(* Logix 5000 AddOnInstructionDefinition export Banner_LM_Param_v4; software revision 33.00 *)

TYPE Banner_IOL_Port_v4 :   // UDT that has all of the data items necessary to communicate with a specific Port on a IO-Link Master
STRUCT
   Port_Controlled : INT;   // Each bit represents a port on an IO-Link Master. Set to 1 to tell AOI to control that port.
   Port_Activate : INT;   // Each bit represents a port on an IO-Link Master. When ON that port will process any commands in queue.
   Port_Read : INT;   // Each bit represents a port on an IO-Link Master. Used to determine when device AOI has requested a Read command.
   Port_Write : INT;   // Each bit represents a port on an IO-Link Master. Used to determine when device AOI has requested a Write command.
   Port_RW_Complete : INT;   // Each bit represents a port on an IO-Link Master. Tells device AOI that Read or Write request has been completed.
   Port_Device_Read : INT;
   Data_Transfer : SINT[190];   // Array to transfer data from IO-Master to device AOIs.
END_STRUCT
END_TYPE

TYPE Banner_LM_RD_v4 :   // UDT that stores the Write Data for a LM.
STRUCT
   Master_Cycle_Time : INT;
   Min_Cycle_Time : INT;
   M_Sequence_Capability : INT;
   IO_Link_Version_ID : INT;
   Process_Data_Input_Length : INT;
   Process_Data_Output_Length : INT;
   Combined_Vendor_ID : DINT;   // IO-Link Vendor ID
   Vendor_ID1 : INT;
   Vendor_ID2 : INT;
   Combined_Device_ID : DINT;   // IO-Link Device ID
   Device_ID1 : INT;
   Device_ID2 : INT;
   Device_ID3 : INT;
   Serial_Number : STRING;
   Teach_State : SINT;   // 0 =IDLE, 1 = SP1 Success, 4 = Wait for Command, 5 = Busy, 7 = Error
   SP1_TP1 : SINT;
   SP2_TP2 : SINT;
   Measurement_Distance : DINT;   // Current measured distance in micrometers.
   Excess_Gain_Percent : DINT;   // Excess gain expressed as a percentage of minimum signal strength.
   Stability : INT;   // 0 = No target exists, 1 = Marginal or multiple peaks, 2 = Stable
   Laser_Fault_Status : INT;   // 0 = Not present, 1 Laser fault present
   Analog_Output_Value : DINT;   // In .01 microAmp increments.
   BDC1_Dual_Mode_Percent : DINT;   // In .01% increments.
   Temperature : INT;
   Last_Taught_Temperature : INT;
   Transducer_Disable_Status : SINT;   // 0 = Active, 1 = Inactive
   All_Time_Run_Time : DINT;   // Run Counter in 1/4 hr increments
   Display_String_Line_1 : STRING;   // String currently being displayed on the LED display of the sensor
   Display_String_Line_2 : STRING;   // String currently being displayed on the LED display of the sensor
   All_Time_Run_Time_Event_Time : DINT;   // Event Time in 1/4 hr increments
END_STRUCT
END_TYPE

TYPE Banner_LM_v4 :   // All of the parameters for a LM.
STRUCT
   Initial_Global_Read : BOOL;   // Determines if all of the IO-Link data has been read into the PLC yet
   Command : INT;   // Value placed in here will activate a read or write to a specifc IO-Link Index
   Read_Data : Banner_LM_RD_v4;   // Read Only Data
   Write_Data : Banner_LM_WD_v4;   // Write Data
   Archive : Banner_LM_WD_v4;   // Archive of Write Data
   Reset : BOOL;   // Resets AOI. This will force a complete parameter read of the sensor.
END_STRUCT
END_TYPE

TYPE Banner_LM_WD_v4 :   // UDT that stores the Write Data for a LM.
STRUCT
   System_Command : INT;   // See IODD file for list of commands that can be activated via the System Command interface
   Parameter_Access_Lock : SINT;   // Write access to all parameters is prohibited while value is 1. Only this parameter can be adjusted when value is 1.
   Data_Storage_Lock : SINT;   // Automatic data storage is disabled when this value is equal to 1. Read access is not affected.
   Local_Parameterization_Lock : SINT;   // Parameterization via local control elements on device is disabled.
   Local_User_Interface_Lock : SINT;   // Operation of local user interface is disabled.
   Teach_Channel : INT;   // 0 = Default, 1 = BDC1, 192 = AO1
   BDC1_Setpoint_SP1 : DINT;   // Switch point value in micrometers. Range: varies depending on sensor.
   BDC1_Setpoint_SP2 : DINT;   // Switch point 2 in window mode only. Range varies depending on sensor.
   BDC1_Swithpoint_Logic : INT;   // 0 = Light Operate, 1 = Dark Operate
   BDC1_BDC_Mode : INT;   // 1 = Switch Mode/Single Point, 2 = Window Mode, 131 = Dual, 132 = Health (LO)/Alarm (DO)
   BDC1_Hysteresis : DINT;   // Should always be 0
   Response_Speed : INT;   // 0 = Fast ms, 1 = Standard, 2 = Medium, 3 = Slow
   Zero_Reference_Location : INT;   // 0 = Near, 1 = Far
   Shift_Zero_Reference_After_Teach : INT;   // 0 = Off, 1 = AutoSet, 2 = SetZero
   Sensor_Lockout : INT;   // 0 =No Lock-out, 1 = Sensor Locked
   Output_Polarity : INT;   // 0 = PNP, 1 = NPN
   IOL_Filter_Time : DINT;   // Time to average IOL process data measurement between updates. Range 0 to 65535 ms.
   Display_Units : SINT;   // 0 = mm, 1 = inches
   Remote_Input_Types : SINT;   // 0 = Type Teach, 1 = Type Laser Enable, 2 = Type Trigger, 3 = Type Sync Master, 4 = Type Sync Slave, 5 = Type Disabled
   Process_Data_Measurement_1_Selection : SINT;   // 0 = Disabled, 1 = Distance Measurement Value, 2 = Displayed Distance Measurement Value, 3 = Analog Output Value, 4 = BDC1 Dual Mode Percent
   Process_Data_Measurement_2_Selection : SINT;   // 0 = Disabled, 1 = Excess Gain, 2 = ExcessGain/10, 3= BDC1 Dual Mode Percent.
   Include_Binary_in_PDI : SINT;   // 0 = Don't include, 1 = Include
   BDC1_Delay_Mode : INT;   // 0 = Disabled, 1 = On - Off Delay, 2 = Off Oneshot, 3 = On Oneshot
   BDC1_Delay_On : DINT;   // Range 0 to 9999 in ms.
   BDC1_Delay_Off : DINT;   // Range 0 to 9999 in ms.
   Swtich_Point_Reference : SINT;   // 0 = Object, 1 = Background, 2= Custom
   User_Teach_Offset : DINT;   // Range -90000 to 90000. User selected teach offset.
   Midpoint_Teach_Window_Size : DINT;   // Range 1000 to 90000. Only used in window mode teach.
   Midpoint_Teach_Offset_Size : DINT;   // Range -90000 to 90000. Offset value that is applied to a midpoint teach.
   BDC_Auto_Thresholding : SINT;   // 0 = On, 1 = Off, 2 = High Speed
   Resettable_Run_Time : DINT;   // Run Counter in 1/4 hr increments
   Resettable_Run_Time_Event_Time : DINT;   // Event Time in 1/4 hour increments
END_STRUCT
END_TYPE

ADD_ON_INSTRUCTION Banner_LM_Param_v4   (* revision 4.1, vendor Banner Engineering *)
// AOI to read and write parameter data to an IO-Link LM.
VAR_IN_OUT
   LM : Banner_LM_v4; {required}
   Port_Data : Banner_IOL_Port_v4; {required}
END_VAR
VAR_INPUT
   Port : INT; {required}
END_VAR
VAR
   Local_Control : DINT; {access None}
   Global_Read_Command_Value : INT; {access None}
   Global_Write_Command_Value : INT; {access None}
   Command_Being_Processed : BOOL; {access None}
   Update_Archive : BOOL; {access None}
   Index_Write_Inprocess : INT; {access None}
   Index_Write_Control : INT; {access None}
   Temp_Excess_Gain : DINT; {access None}
   Inprocess_Index : DINT; {access None}
END_VAR

ROUTINE Logic   (* ladder *)
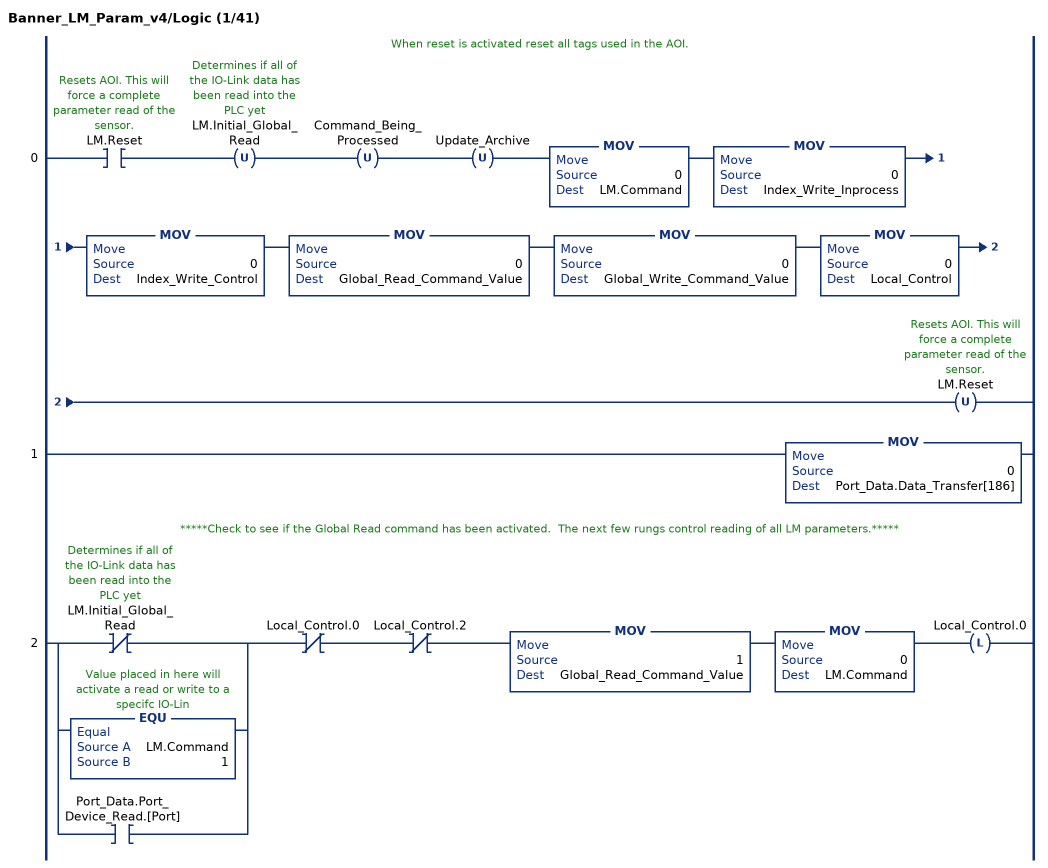
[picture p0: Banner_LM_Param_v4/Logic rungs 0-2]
   // When reset is activated reset all tags used in the AOI.
   0: XIC(LM.Reset)OTU(LM.Initial_Global_Read)OTU(Command_Being_Processed)OTU(Update_Archive)MOV(0,LM.Command)MOV(0,Index_Write_Inprocess)MOV(0,Index_Write_Control)MOV(0,Global_Read_Command_Value)MOV(0,Global_Write_Command_Value)MOV(0,Local_Control)OTU(LM.Reset);
   1: MOV(0,Port_Data.Data_Transfer[186]);
   // *****Check to see if the Global Read command has been activated.  The next few rungs control reading of all LM parameters.*****
   2: [XIO(LM.Initial_Global_Read) ,EQU(LM.Command,1) ,XIC(Port_Data.Port_Device_Read.[Port]) ]XIO(Local_Control.0)XIO(Local_Control.2)MOV(1,Global_Read_Command_Value)MOV(0,LM.Command)OTL(Local_Control.0);
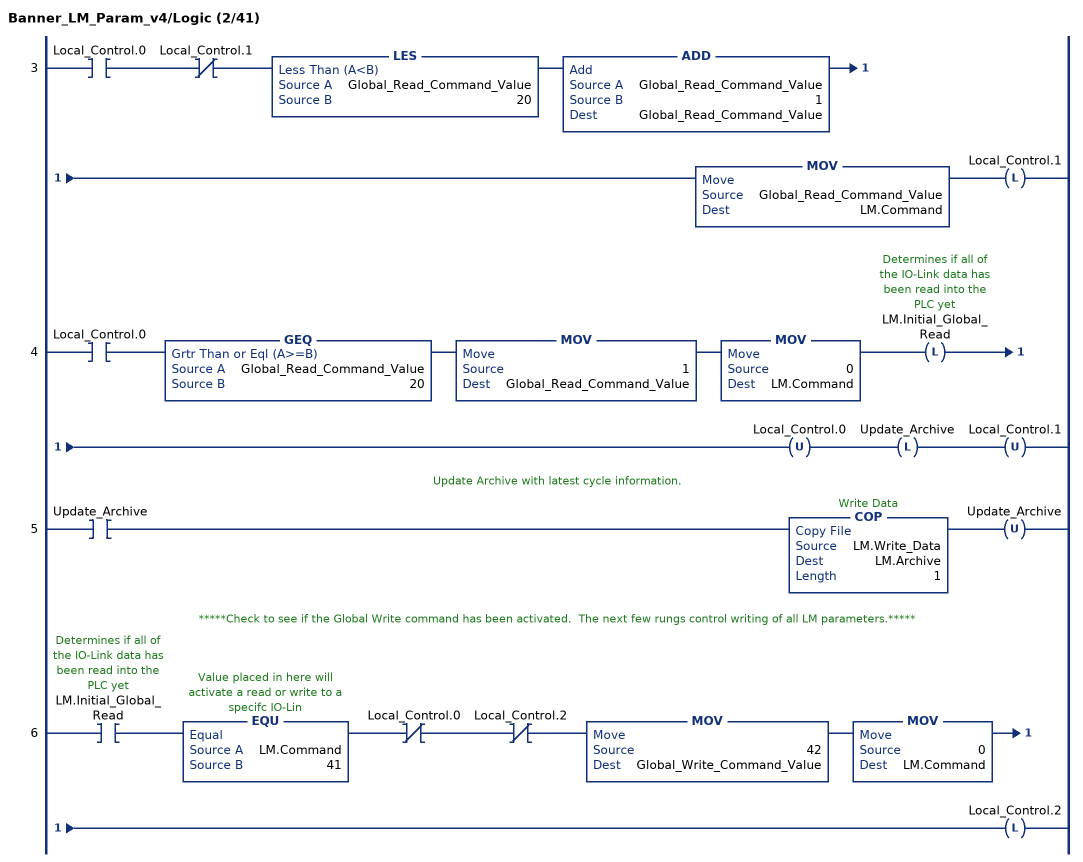
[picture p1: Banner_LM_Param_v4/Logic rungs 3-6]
   3: XIC(Local_Control.0)XIO(Local_Control.1)LES(Global_Read_Command_Value,20)ADD(Global_Read_Command_Value,1,Global_Read_Command_Value)MOV(Global_Read_Command_Value,LM.Command)OTL(Local_Control.1);
   4: XIC(Local_Control.0)GEQ(Global_Read_Command_Value,20)MOV(1,Global_Read_Command_Value)MOV(0,LM.Command)OTL(LM.Initial_Global_Read)OTU(Local_Control.0)OTL(Update_Archive)OTU(Local_Control.1);
   // Update Archive with latest cycle information.
   5: XIC(Update_Archive)COP(LM.Write_Data,LM.Archive,1)OTU(Update_Archive);
   // *****Check to see if the Global Write command has been activated.  The next few rungs control writing of all LM parameters.*****
   6: XIC(LM.Initial_Global_Read)EQU(LM.Command,41)XIO(Local_Control.0)XIO(Local_Control.2)MOV(42,Global_Write_Command_Value)MOV(0,LM.Command)OTL(Local_Control.2);
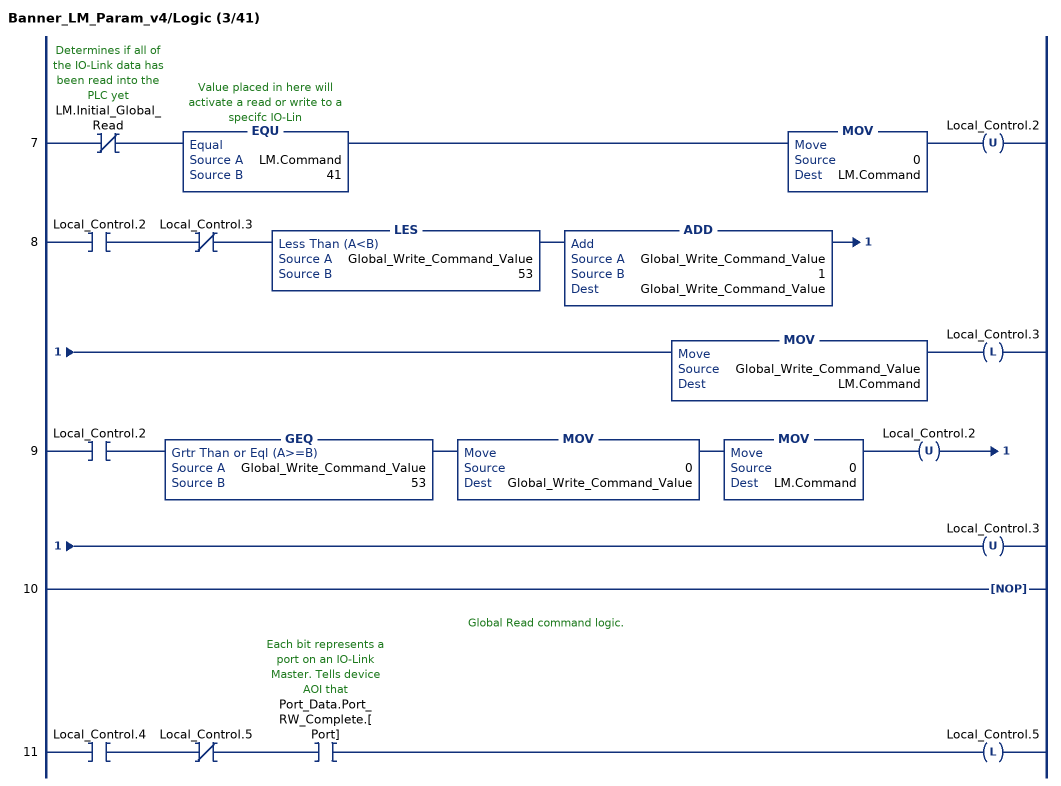
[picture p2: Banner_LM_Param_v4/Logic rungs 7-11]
   7: XIO(LM.Initial_Global_Read)EQU(LM.Command,41)MOV(0,LM.Command)OTU(Local_Control.2);
   8: XIC(Local_Control.2)XIO(Local_Control.3)LES(Global_Write_Command_Value,53)ADD(Global_Write_Command_Value,1,Global_Write_Command_Value)MOV(Global_Write_Command_Value,LM.Command)OTL(Local_Control.3);
   9: XIC(Local_Control.2)GEQ(Global_Write_Command_Value,53)MOV(0,Global_Write_Command_Value)MOV(0,LM.Command)OTU(Local_Control.2)OTU(Local_Control.3);
   10: NOP();
   // Global Read command logic.
   11: XIC(Local_Control.4)XIO(Local_Control.5)XIC(Port_Data.Port_RW_Complete.[Port])OTL(Local_Control.5);
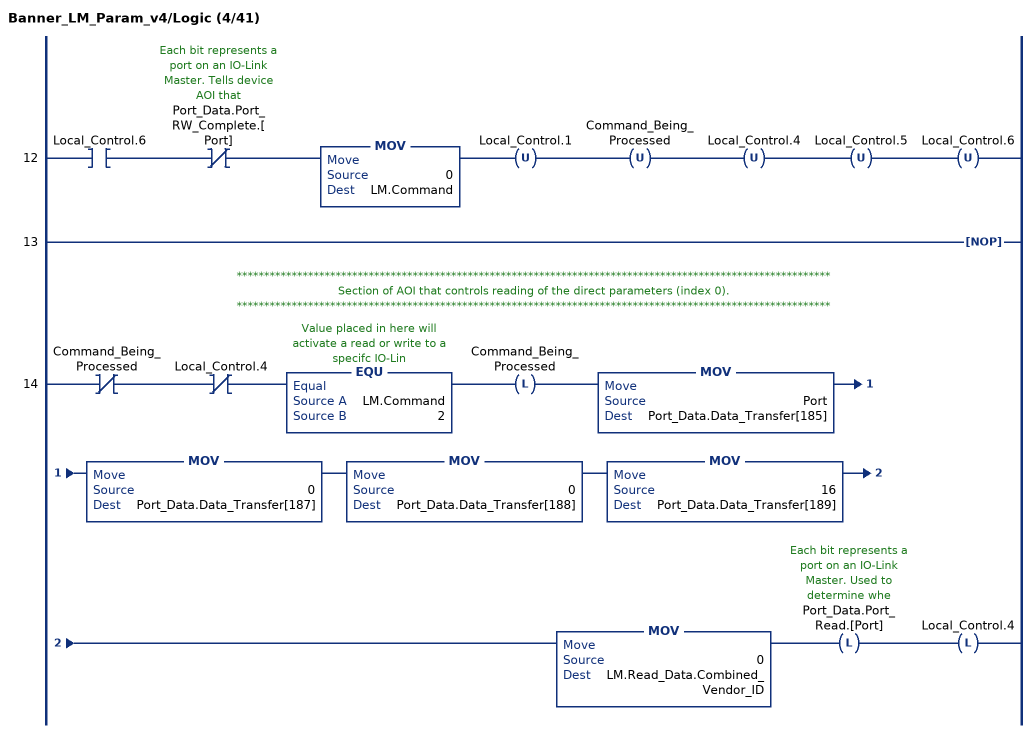
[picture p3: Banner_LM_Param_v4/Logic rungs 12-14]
   12: XIC(Local_Control.6)XIO(Port_Data.Port_RW_Complete.[Port])MOV(0,LM.Command)OTU(Local_Control.1)OTU(Command_Being_Processed)OTU(Local_Control.4)OTU(Local_Control.5)OTU(Local_Control.6);
   13: NOP();
   // ************************************************************************************************************
   // Section of AOI that controls reading of the direct parameters (index 0).
   // ************************************************************************************************************
   14: XIO(Command_Being_Processed)XIO(Local_Control.4)EQU(LM.Command,2)OTL(Command_Being_Processed)MOV(Port,Port_Data.Data_Transfer[185])MOV(0,Port_Data.Data_Transfer[187])MOV(0,Port_Data.Data_Transfer[188])MOV(16,Port_Data.Data_Transfer[189])MOV(0,LM.Read_Data.Combined_Vendor_ID)OTL(Port_Data.Port_Read.[Port])OTL(Local_Control.4);
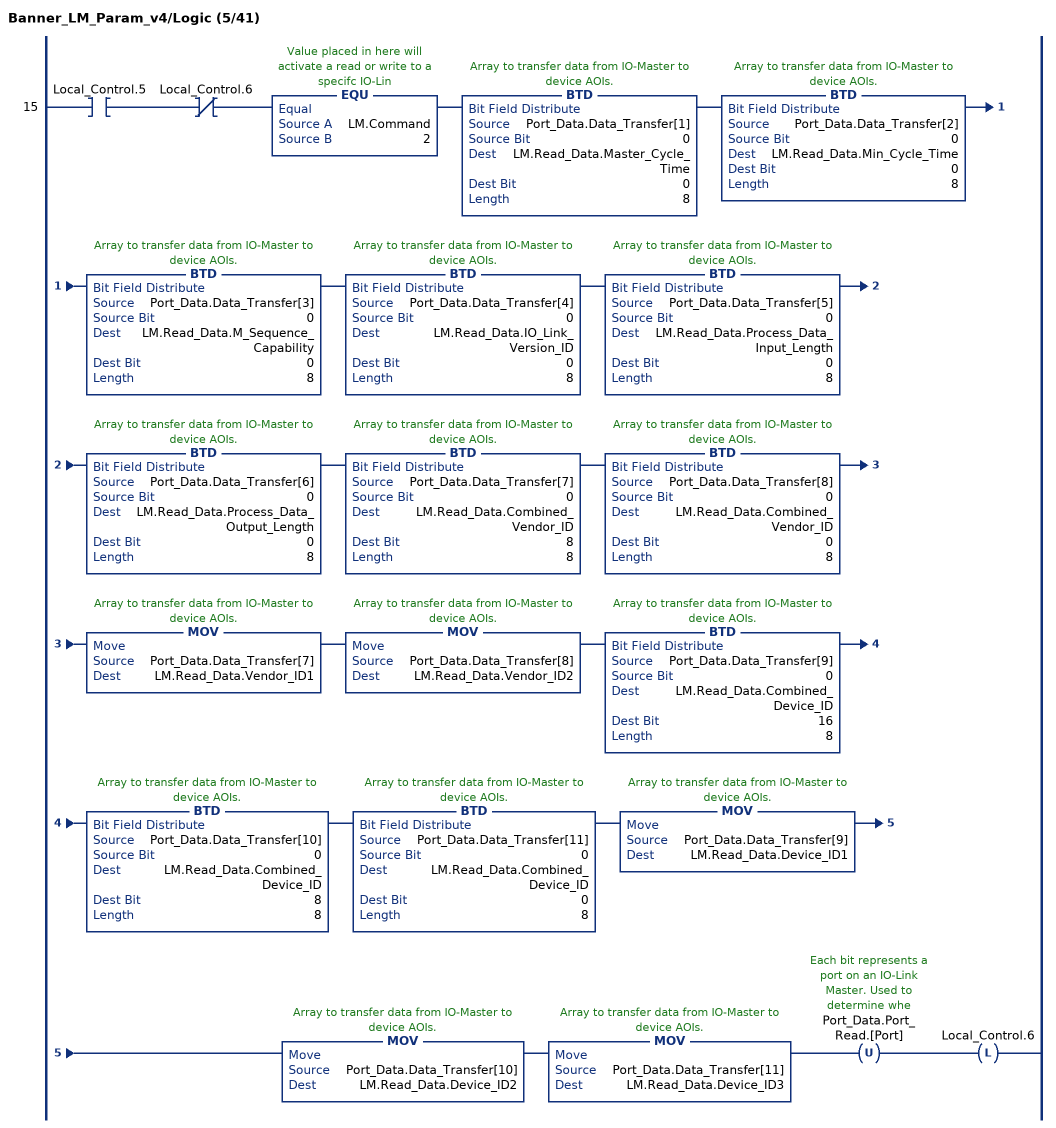
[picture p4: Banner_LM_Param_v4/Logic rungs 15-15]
   15: XIC(Local_Control.5)XIO(Local_Control.6)EQU(LM.Command,2)BTD(Port_Data.Data_Transfer[1],0,LM.Read_Data.Master_Cycle_Time,0,8)BTD(Port_Data.Data_Transfer[2],0,LM.Read_Data.Min_Cycle_Time,0,8)BTD(Port_Data.Data_Transfer[3],0,LM.Read_Data.M_Sequence_Capability,0,8)BTD(Port_Data.Data_Transfer[4],0,LM.Read_Data.IO_Link_Version_ID,0,8)BTD(Port_Data.Data_Transfer[5],0,LM.Read_Data.Process_Data_Input_Length,0,8)BTD(Port_Data.Data_Transfer[6],0,LM.Read_Data.Process_Data_Output_Length,0,8)BTD(Port_Data.Data_Transfer[7],0,LM.Read_Data.Combined_Vendor_ID,8,8)BTD(Port_Data.Data_Transfer[8],0,LM.Read_Data.Combined_Vendor_ID,0,8)MOV(Port_Data.Data_Transfer[7],LM.Read_Data.Vendor_ID1)MOV(Port_Data.Data_Transfer[8],LM.Read_Data.Vendor_ID2)BTD(Port_Data.Data_Transfer[9],0,LM.Read_Data.Combined_Device_ID,16,8)BTD(Port_Data.Data_Transfer[10],0,LM.Read_Data.Combined_Device_ID,8,8)BTD(Port_Data.Data_Transfer[11],0,LM.Read_Data.Combined_Device_ID,0,8)MOV(Port_Data.Data_Transfer[9],LM.Read_Data.Device_ID1)MOV(Port_Data.Data_Transfer[10],LM.Read_Data.Device_ID2)MOV(Port_Data.Data_Transfer[11],LM.Read_Data.Device_ID3)OTU(Port_Data.Port_Read.[Port])OTL(Local_Control.6);
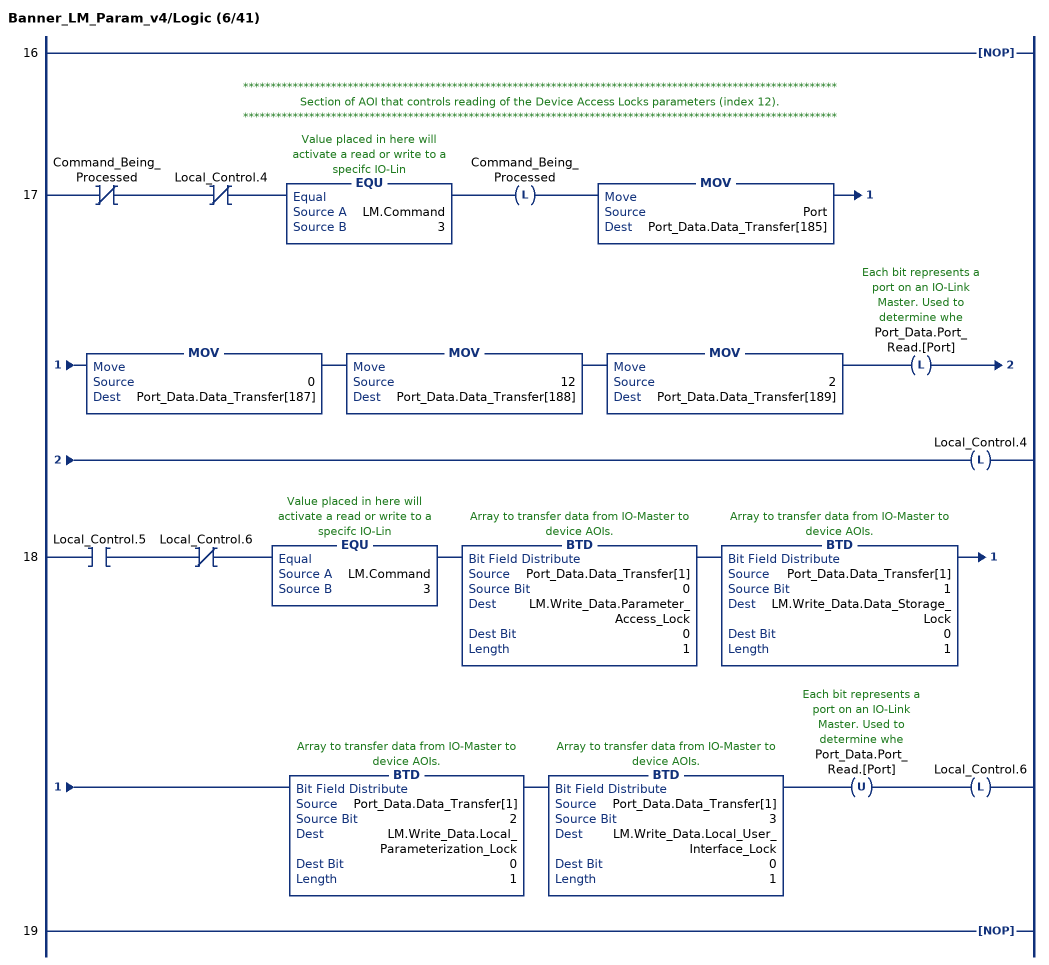
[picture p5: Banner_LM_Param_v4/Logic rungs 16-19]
   16: NOP();
   // ************************************************************************************************************
   // Section of AOI that controls reading of the Device Access Locks parameters (index 12).
   // ************************************************************************************************************
   17: XIO(Command_Being_Processed)XIO(Local_Control.4)EQU(LM.Command,3)OTL(Command_Being_Processed)MOV(Port,Port_Data.Data_Transfer[185])MOV(0,Port_Data.Data_Transfer[187])MOV(12,Port_Data.Data_Transfer[188])MOV(2,Port_Data.Data_Transfer[189])OTL(Port_Data.Port_Read.[Port])OTL(Local_Control.4);
   18: XIC(Local_Control.5)XIO(Local_Control.6)EQU(LM.Command,3)BTD(Port_Data.Data_Transfer[1],0,LM.Write_Data.Parameter_Access_Lock,0,1)BTD(Port_Data.Data_Transfer[1],1,LM.Write_Data.Data_Storage_Lock,0,1)BTD(Port_Data.Data_Transfer[1],2,LM.Write_Data.Local_Parameterization_Lock,0,1)BTD(Port_Data.Data_Transfer[1],3,LM.Write_Data.Local_User_Interface_Lock,0,1)OTU(Port_Data.Port_Read.[Port])OTL(Local_Control.6);
   19: NOP();
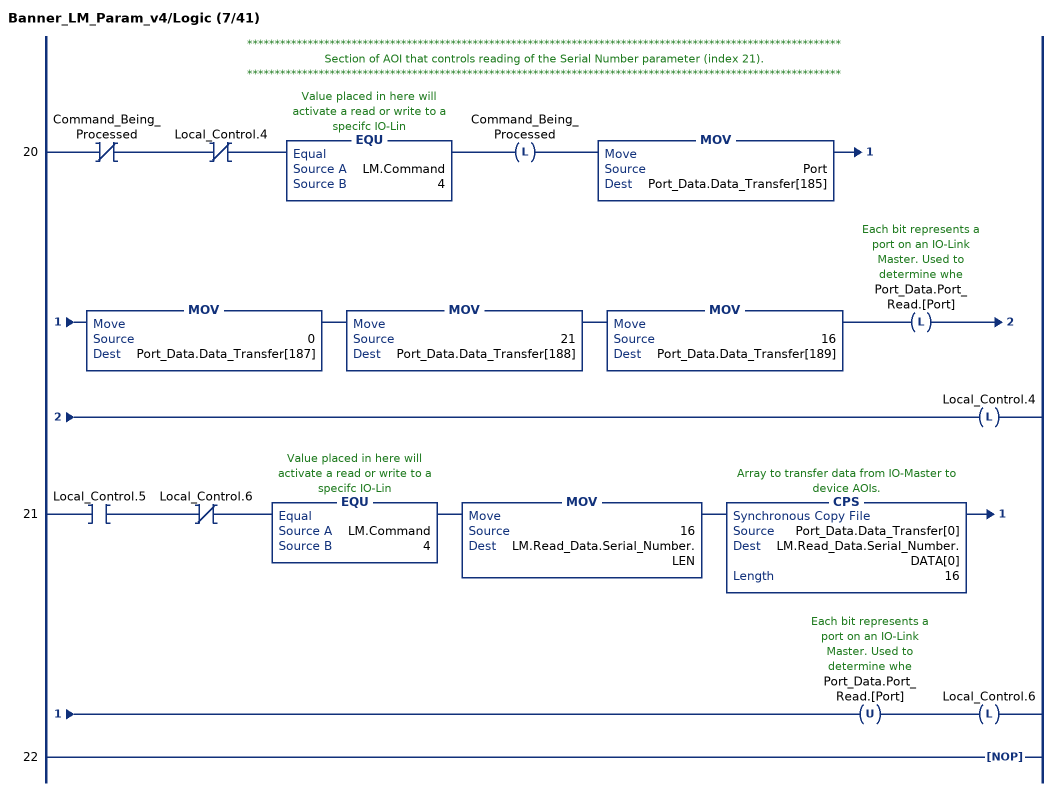
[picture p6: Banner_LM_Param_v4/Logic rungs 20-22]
   // ************************************************************************************************************
   // Section of AOI that controls reading of the Serial Number parameter (index 21).
   // ************************************************************************************************************
   20: XIO(Command_Being_Processed)XIO(Local_Control.4)EQU(LM.Command,4)OTL(Command_Being_Processed)MOV(Port,Port_Data.Data_Transfer[185])MOV(0,Port_Data.Data_Transfer[187])MOV(21,Port_Data.Data_Transfer[188])MOV(16,Port_Data.Data_Transfer[189])OTL(Port_Data.Port_Read.[Port])OTL(Local_Control.4);
   21: XIC(Local_Control.5)XIO(Local_Control.6)EQU(LM.Command,4)MOV(16,LM.Read_Data.Serial_Number.LEN)CPS(Port_Data.Data_Transfer[0],LM.Read_Data.Serial_Number.DATA[0],16)OTU(Port_Data.Port_Read.[Port])OTL(Local_Control.6);
   22: NOP();
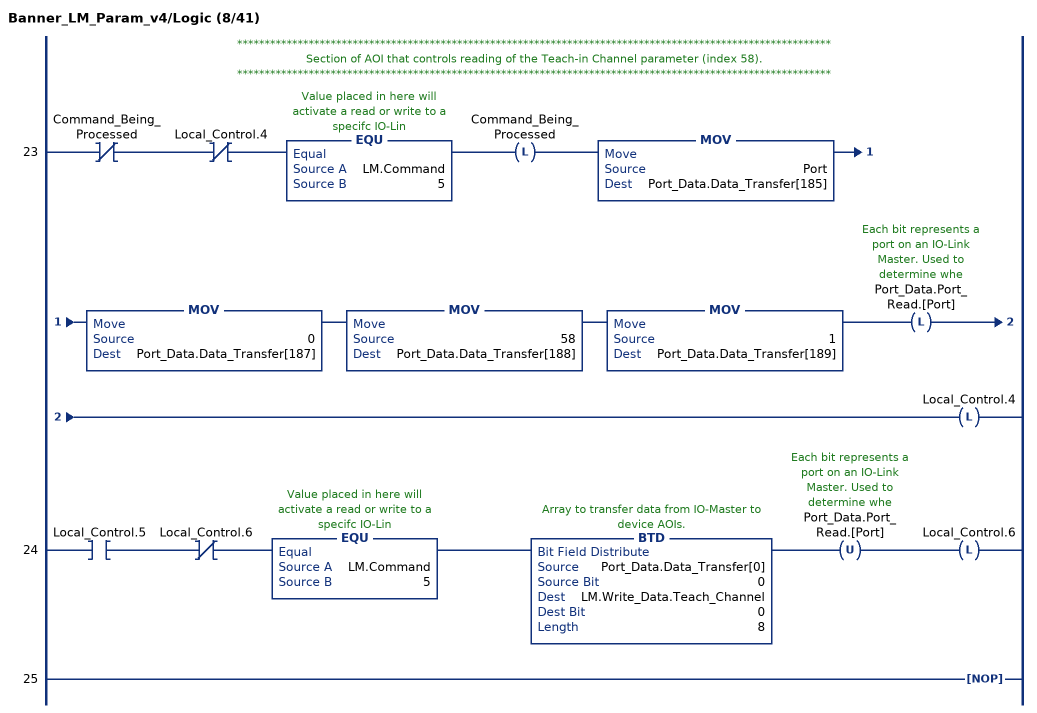
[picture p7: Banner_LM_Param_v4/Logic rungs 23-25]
   // ************************************************************************************************************
   // Section of AOI that controls reading of the Teach-in Channel parameter (index 58).
   // ************************************************************************************************************
   23: XIO(Command_Being_Processed)XIO(Local_Control.4)EQU(LM.Command,5)OTL(Command_Being_Processed)MOV(Port,Port_Data.Data_Transfer[185])MOV(0,Port_Data.Data_Transfer[187])MOV(58,Port_Data.Data_Transfer[188])MOV(1,Port_Data.Data_Transfer[189])OTL(Port_Data.Port_Read.[Port])OTL(Local_Control.4);
   24: XIC(Local_Control.5)XIO(Local_Control.6)EQU(LM.Command,5)BTD(Port_Data.Data_Transfer[0],0,LM.Write_Data.Teach_Channel,0,8)OTU(Port_Data.Port_Read.[Port])OTL(Local_Control.6);
   25: NOP();
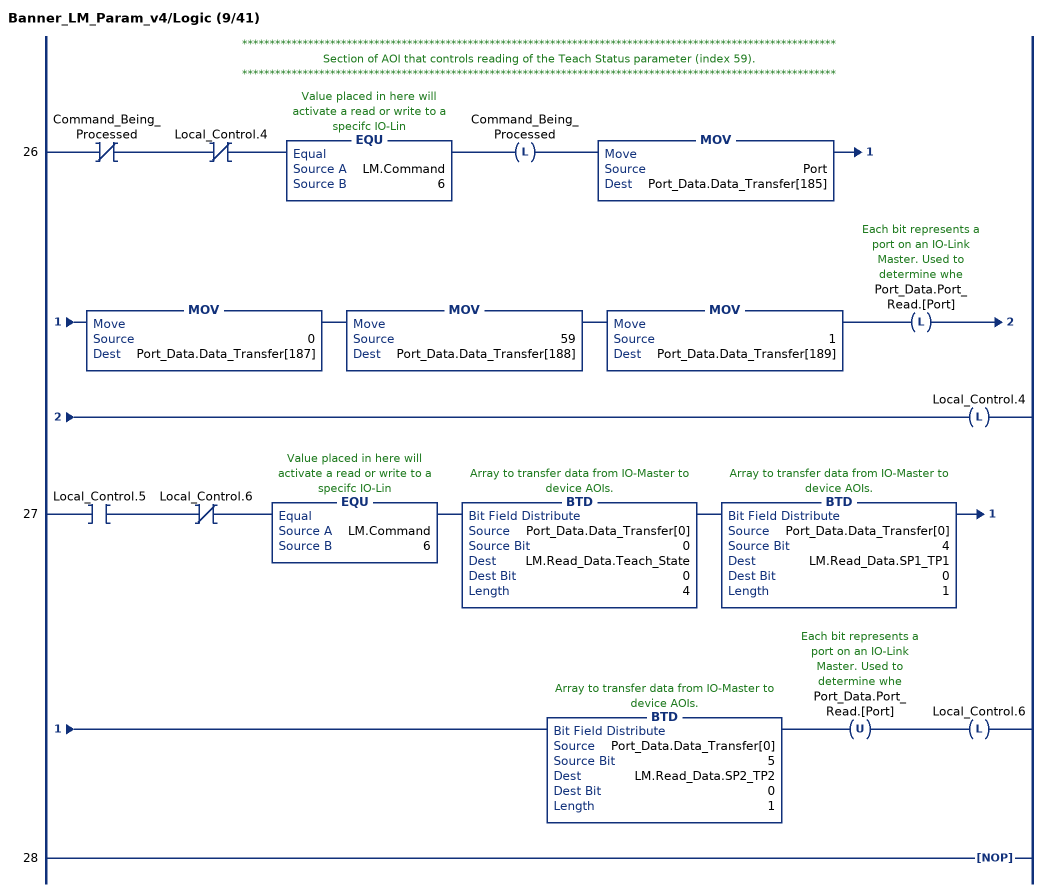
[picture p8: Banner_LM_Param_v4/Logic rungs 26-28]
   // ************************************************************************************************************
   // Section of AOI that controls reading of the Teach Status parameter (index 59).
   // ************************************************************************************************************
   26: XIO(Command_Being_Processed)XIO(Local_Control.4)EQU(LM.Command,6)OTL(Command_Being_Processed)MOV(Port,Port_Data.Data_Transfer[185])MOV(0,Port_Data.Data_Transfer[187])MOV(59,Port_Data.Data_Transfer[188])MOV(1,Port_Data.Data_Transfer[189])OTL(Port_Data.Port_Read.[Port])OTL(Local_Control.4);
   27: XIC(Local_Control.5)XIO(Local_Control.6)EQU(LM.Command,6)BTD(Port_Data.Data_Transfer[0],0,LM.Read_Data.Teach_State,0,4)BTD(Port_Data.Data_Transfer[0],4,LM.Read_Data.SP1_TP1,0,1)BTD(Port_Data.Data_Transfer[0],5,LM.Read_Data.SP2_TP2,0,1)OTU(Port_Data.Port_Read.[Port])OTL(Local_Control.6);
   28: NOP();
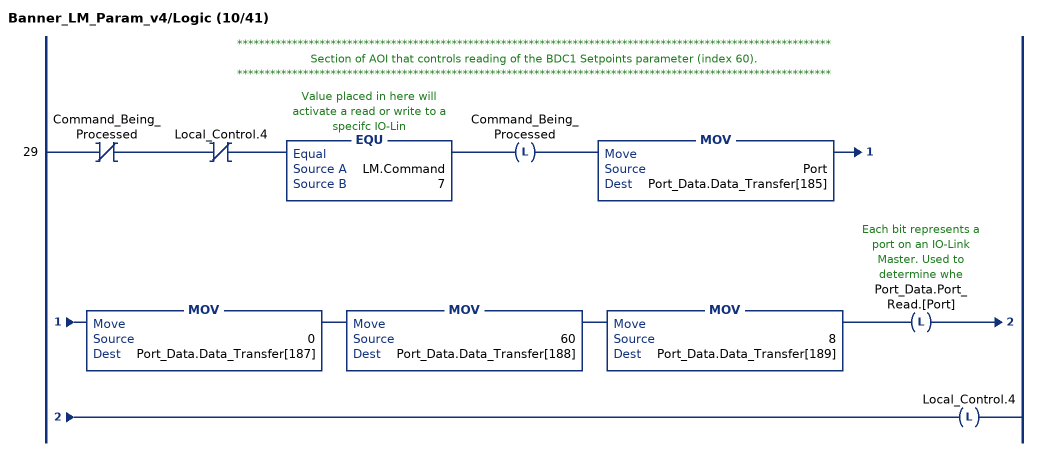
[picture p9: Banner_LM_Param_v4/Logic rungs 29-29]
   // ************************************************************************************************************
   // Section of AOI that controls reading of the BDC1 Setpoints parameter (index 60).
   // ************************************************************************************************************
   29: XIO(Command_Being_Processed)XIO(Local_Control.4)EQU(LM.Command,7)OTL(Command_Being_Processed)MOV(Port,Port_Data.Data_Transfer[185])MOV(0,Port_Data.Data_Transfer[187])MOV(60,Port_Data.Data_Transfer[188])MOV(8,Port_Data.Data_Transfer[189])OTL(Port_Data.Port_Read.[Port])OTL(Local_Control.4);
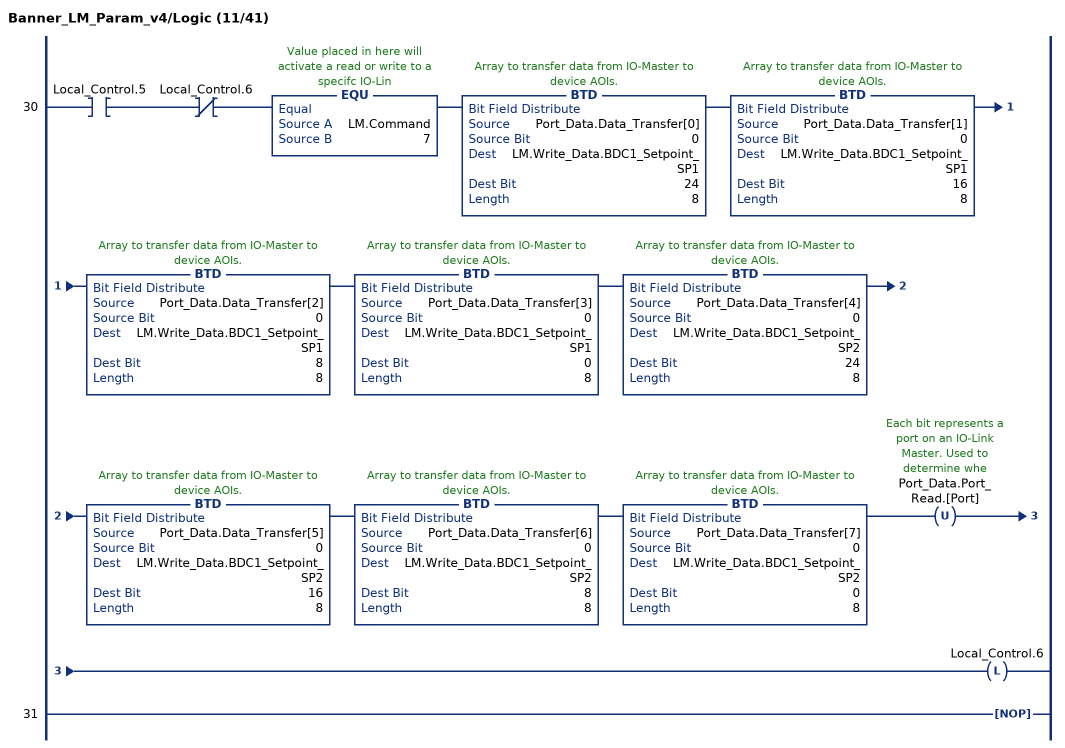
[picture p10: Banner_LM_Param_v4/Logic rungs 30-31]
   30: XIC(Local_Control.5)XIO(Local_Control.6)EQU(LM.Command,7)BTD(Port_Data.Data_Transfer[0],0,LM.Write_Data.BDC1_Setpoint_SP1,24,8)BTD(Port_Data.Data_Transfer[1],0,LM.Write_Data.BDC1_Setpoint_SP1,16,8)BTD(Port_Data.Data_Transfer[2],0,LM.Write_Data.BDC1_Setpoint_SP1,8,8)BTD(Port_Data.Data_Transfer[3],0,LM.Write_Data.BDC1_Setpoint_SP1,0,8)BTD(Port_Data.Data_Transfer[4],0,LM.Write_Data.BDC1_Setpoint_SP2,24,8)BTD(Port_Data.Data_Transfer[5],0,LM.Write_Data.BDC1_Setpoint_SP2,16,8)BTD(Port_Data.Data_Transfer[6],0,LM.Write_Data.BDC1_Setpoint_SP2,8,8)BTD(Port_Data.Data_Transfer[7],0,LM.Write_Data.BDC1_Setpoint_SP2,0,8)OTU(Port_Data.Port_Read.[Port])OTL(Local_Control.6);
   31: NOP();
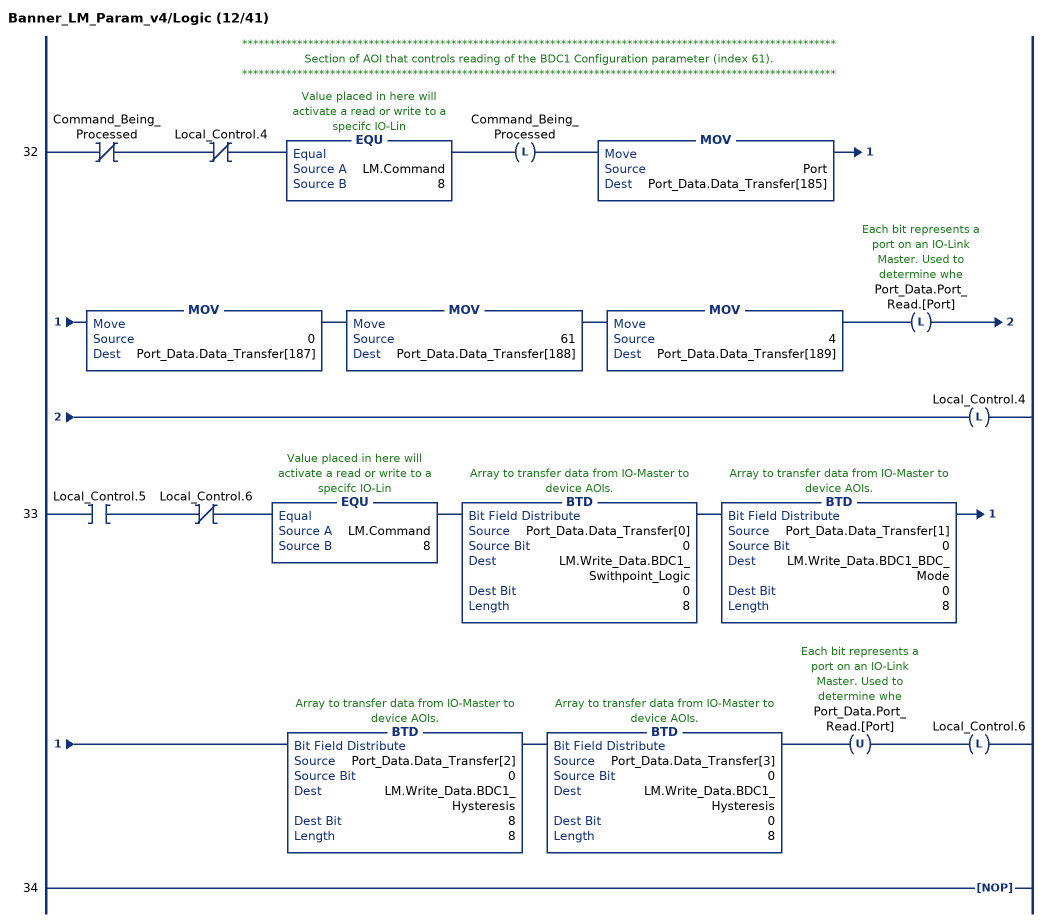
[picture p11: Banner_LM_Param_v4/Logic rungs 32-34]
   // ************************************************************************************************************
   // Section of AOI that controls reading of the BDC1 Configuration parameter (index 61).
   // ************************************************************************************************************
   32: XIO(Command_Being_Processed)XIO(Local_Control.4)EQU(LM.Command,8)OTL(Command_Being_Processed)MOV(Port,Port_Data.Data_Transfer[185])MOV(0,Port_Data.Data_Transfer[187])MOV(61,Port_Data.Data_Transfer[188])MOV(4,Port_Data.Data_Transfer[189])OTL(Port_Data.Port_Read.[Port])OTL(Local_Control.4);
   33: XIC(Local_Control.5)XIO(Local_Control.6)EQU(LM.Command,8)BTD(Port_Data.Data_Transfer[0],0,LM.Write_Data.BDC1_Swithpoint_Logic,0,8)BTD(Port_Data.Data_Transfer[1],0,LM.Write_Data.BDC1_BDC_Mode,0,8)BTD(Port_Data.Data_Transfer[2],0,LM.Write_Data.BDC1_Hysteresis,8,8)BTD(Port_Data.Data_Transfer[3],0,LM.Write_Data.BDC1_Hysteresis,0,8)OTU(Port_Data.Port_Read.[Port])OTL(Local_Control.6);
   34: NOP();
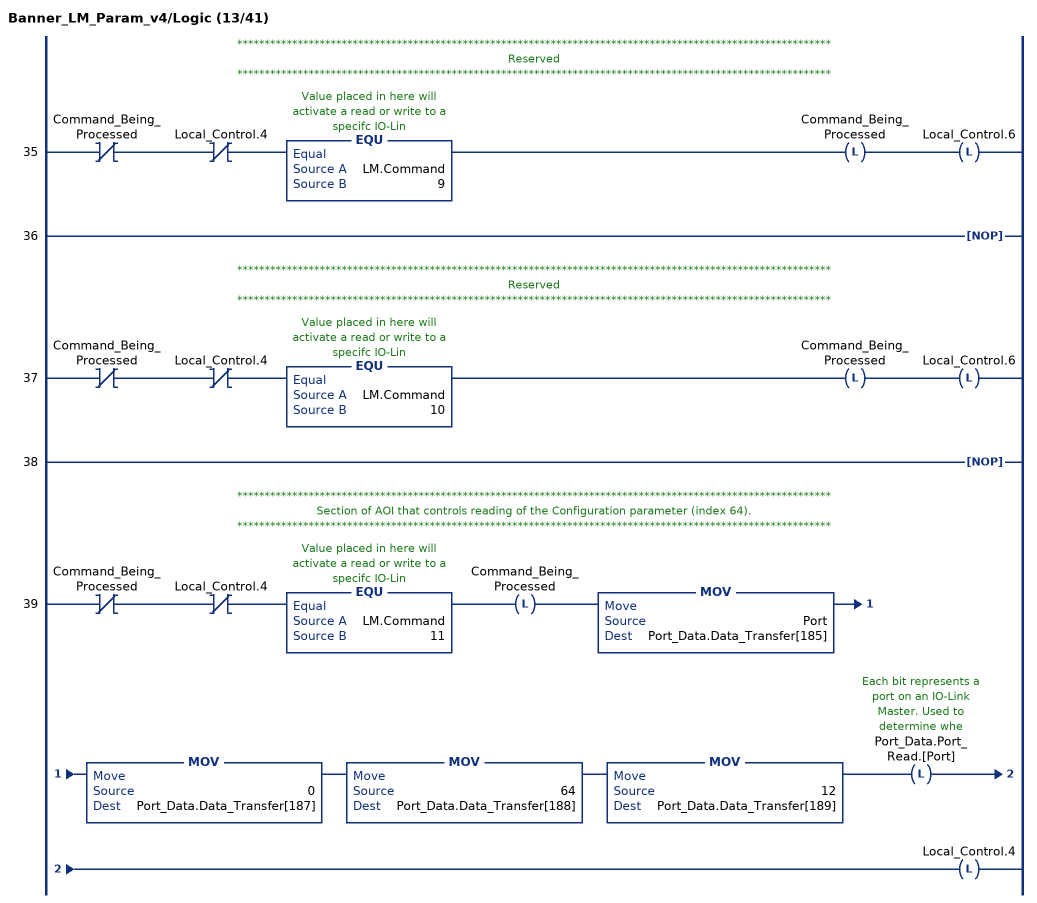
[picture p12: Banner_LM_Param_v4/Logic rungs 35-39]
   // ************************************************************************************************************
   // Reserved
   // ************************************************************************************************************
   35: XIO(Command_Being_Processed)XIO(Local_Control.4)EQU(LM.Command,9)OTL(Command_Being_Processed)OTL(Local_Control.6);
   36: NOP();
   // ************************************************************************************************************
   // Reserved
   // ************************************************************************************************************
   37: XIO(Command_Being_Processed)XIO(Local_Control.4)EQU(LM.Command,10)OTL(Command_Being_Processed)OTL(Local_Control.6);
   38: NOP();
   // ************************************************************************************************************
   // Section of AOI that controls reading of the Configuration parameter (index 64).
   // ************************************************************************************************************
   39: XIO(Command_Being_Processed)XIO(Local_Control.4)EQU(LM.Command,11)OTL(Command_Being_Processed)MOV(Port,Port_Data.Data_Transfer[185])MOV(0,Port_Data.Data_Transfer[187])MOV(64,Port_Data.Data_Transfer[188])MOV(12,Port_Data.Data_Transfer[189])OTL(Port_Data.Port_Read.[Port])OTL(Local_Control.4);
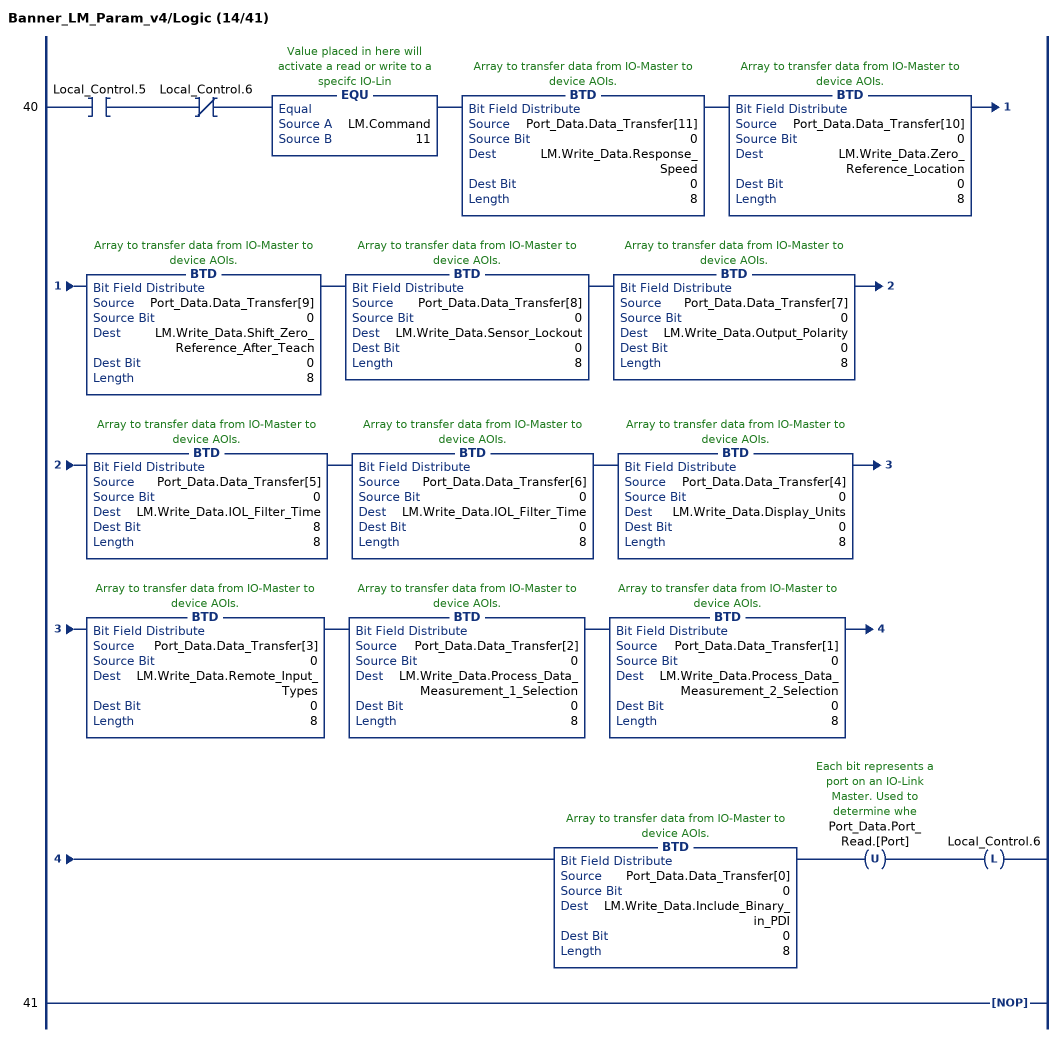
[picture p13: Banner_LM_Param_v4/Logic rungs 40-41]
   40: XIC(Local_Control.5)XIO(Local_Control.6)EQU(LM.Command,11)BTD(Port_Data.Data_Transfer[11],0,LM.Write_Data.Response_Speed,0,8)BTD(Port_Data.Data_Transfer[10],0,LM.Write_Data.Zero_Reference_Location,0,8)BTD(Port_Data.Data_Transfer[9],0,LM.Write_Data.Shift_Zero_Reference_After_Teach,0,8)BTD(Port_Data.Data_Transfer[8],0,LM.Write_Data.Sensor_Lockout,0,8)BTD(Port_Data.Data_Transfer[7],0,LM.Write_Data.Output_Polarity,0,8)BTD(Port_Data.Data_Transfer[5],0,LM.Write_Data.IOL_Filter_Time,8,8)BTD(Port_Data.Data_Transfer[6],0,LM.Write_Data.IOL_Filter_Time,0,8)BTD(Port_Data.Data_Transfer[4],0,LM.Write_Data.Display_Units,0,8)BTD(Port_Data.Data_Transfer[3],0,LM.Write_Data.Remote_Input_Types,0,8)BTD(Port_Data.Data_Transfer[2],0,LM.Write_Data.Process_Data_Measurement_1_Selection,0,8)BTD(Port_Data.Data_Transfer[1],0,LM.Write_Data.Process_Data_Measurement_2_Selection,0,8)BTD(Port_Data.Data_Transfer[0],0,LM.Write_Data.Include_Binary_in_PDI,0,8)OTU(Port_Data.Port_Read.[Port])OTL(Local_Control.6);
   41: NOP();
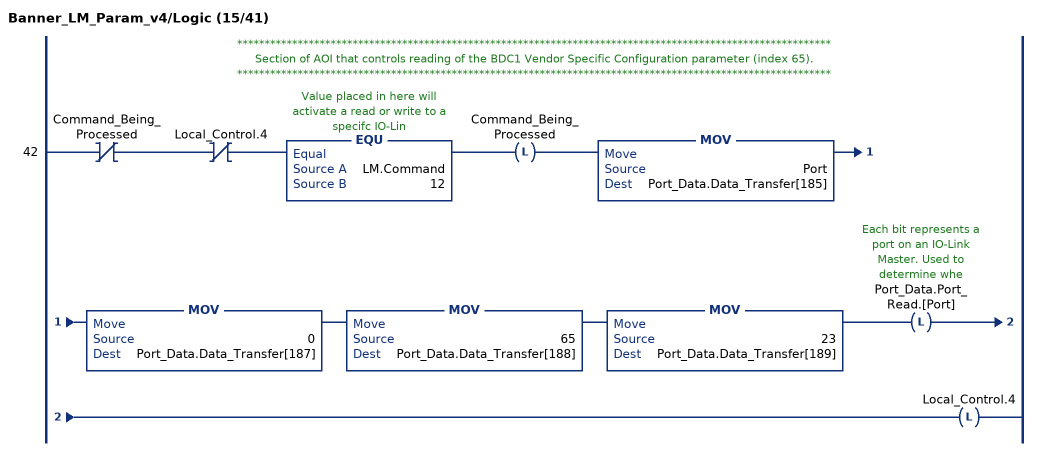
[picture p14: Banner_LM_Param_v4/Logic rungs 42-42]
   // ************************************************************************************************************
   // Section of AOI that controls reading of the BDC1 Vendor Specific Configuration parameter (index 65).
   // ************************************************************************************************************
   42: XIO(Command_Being_Processed)XIO(Local_Control.4)EQU(LM.Command,12)OTL(Command_Being_Processed)MOV(Port,Port_Data.Data_Transfer[185])MOV(0,Port_Data.Data_Transfer[187])MOV(65,Port_Data.Data_Transfer[188])MOV(23,Port_Data.Data_Transfer[189])OTL(Port_Data.Port_Read.[Port])OTL(Local_Control.4);
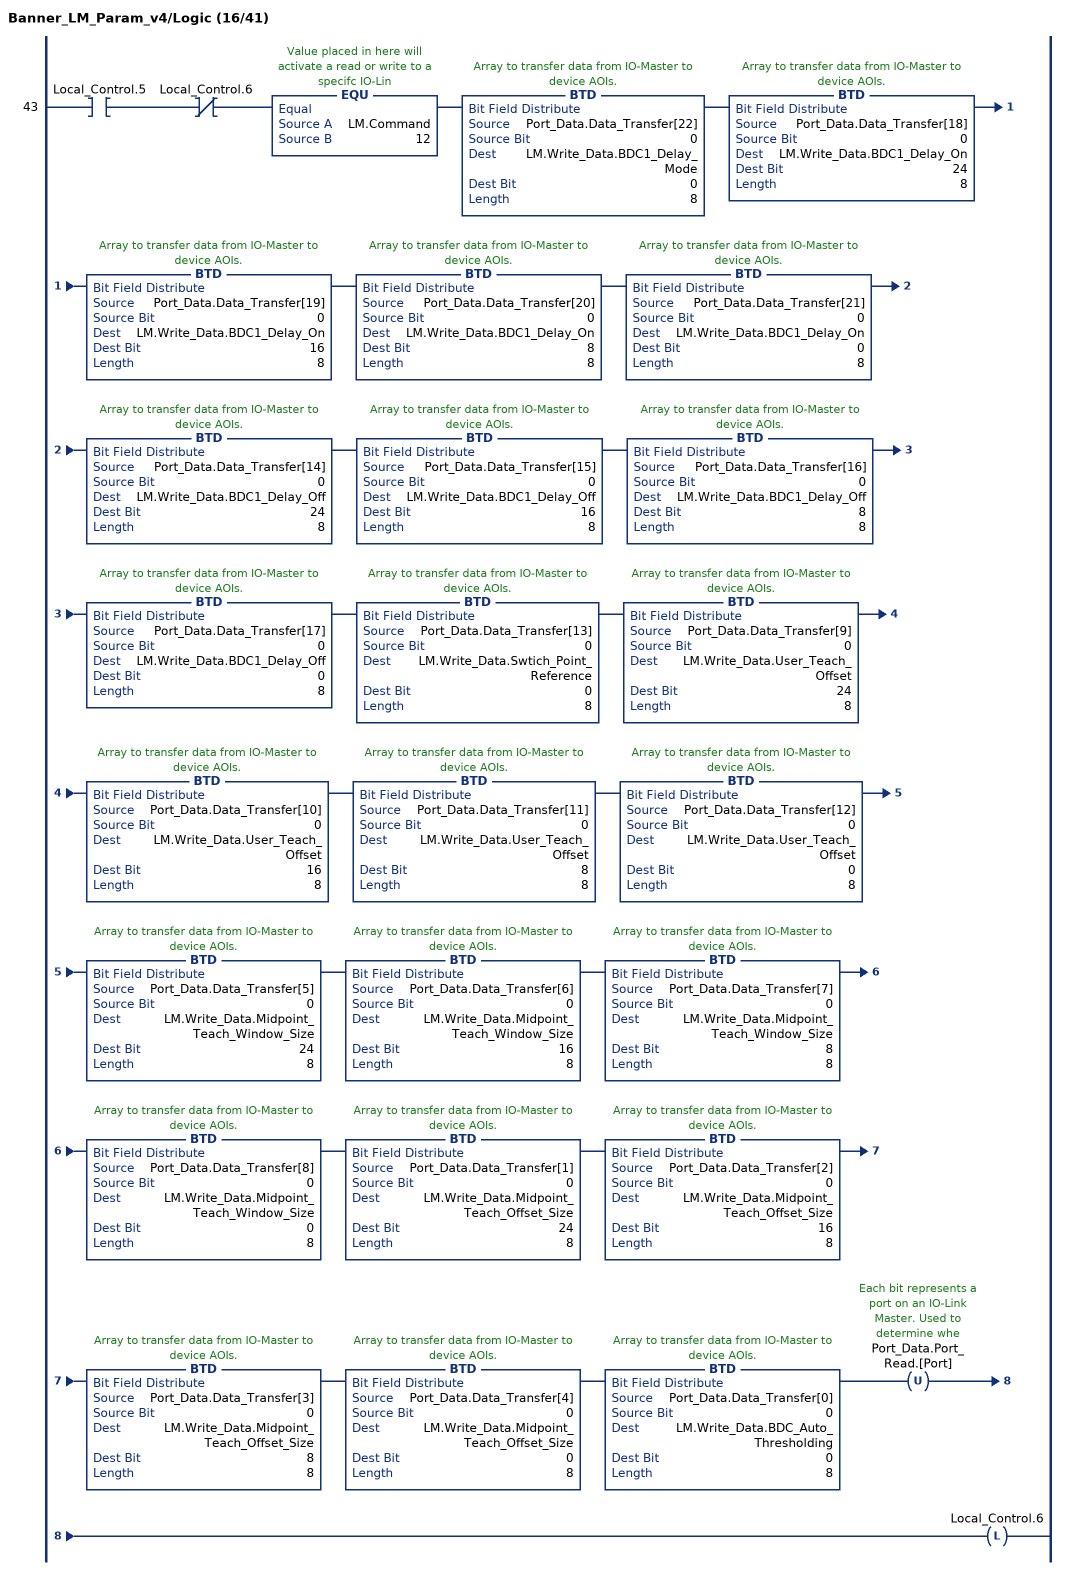
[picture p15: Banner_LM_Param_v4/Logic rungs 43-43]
   43: XIC(Local_Control.5)XIO(Local_Control.6)EQU(LM.Command,12)BTD(Port_Data.Data_Transfer[22],0,LM.Write_Data.BDC1_Delay_Mode,0,8)BTD(Port_Data.Data_Transfer[18],0,LM.Write_Data.BDC1_Delay_On,24,8)BTD(Port_Data.Data_Transfer[19],0,LM.Write_Data.BDC1_Delay_On,16,8)BTD(Port_Data.Data_Transfer[20],0,LM.Write_Data.BDC1_Delay_On,8,8)BTD(Port_Data.Data_Transfer[21],0,LM.Write_Data.BDC1_Delay_On,0,8)BTD(Port_Data.Data_Transfer[14],0,LM.Write_Data.BDC1_Delay_Off,24,8)BTD(Port_Data.Data_Transfer[15],0,LM.Write_Data.BDC1_Delay_Off,16,8)BTD(Port_Data.Data_Transfer[16],0,LM.Write_Data.BDC1_Delay_Off,8,8)BTD(Port_Data.Data_Transfer[17],0,LM.Write_Data.BDC1_Delay_Off,0,8)BTD(Port_Data.Data_Transfer[13],0,LM.Write_Data.Swtich_Point_Reference,0,8)BTD(Port_Data.Data_Transfer[9],0,LM.Write_Data.User_Teach_Offset,24,8)BTD(Port_Data.Data_Transfer[10],0,LM.Write_Data.User_Teach_Offset,16,8)BTD(Port_Data.Data_Transfer[11],0,LM.Write_Data.User_Teach_Offset,8,8)BTD(Port_Data.Data_Transfer[12],0,LM.Write_Data.User_Teach_Offset,0,8)BTD(Port_Data.Data_Transfer[5],0,LM.Write_Data.Midpoint_Teach_Window_Size,24,8)BTD(Port_Data.Data_Transfer[6],0,LM.Write_Data.Midpoint_Teach_Window_Size,16,8)BTD(Port_Data.Data_Transfer[7],0,LM.Write_Data.Midpoint_Teach_Window_Size,8,8)BTD(Port_Data.Data_Transfer[8],0,LM.Write_Data.Midpoint_Teach_Window_Size,0,8)BTD(Port_Data.Data_Transfer[1],0,LM.Write_Data.Midpoint_Teach_Offset_Size,24,8)BTD(Port_Data.Data_Transfer[2],0,LM.Write_Data.Midpoint_Teach_Offset_Size,16,8)BTD(Port_Data.Data_Transfer[3],0,LM.Write_Data.Midpoint_Teach_Offset_Size,8,8)BTD(Port_Data.Data_Transfer[4],0,LM.Write_Data.Midpoint_Teach_Offset_Size,0,8)BTD(Port_Data.Data_Transfer[0],0,LM.Write_Data.BDC_Auto_Thresholding,0,8)OTU(Port_Data.Port_Read.[Port])OTL(Local_Control.6);
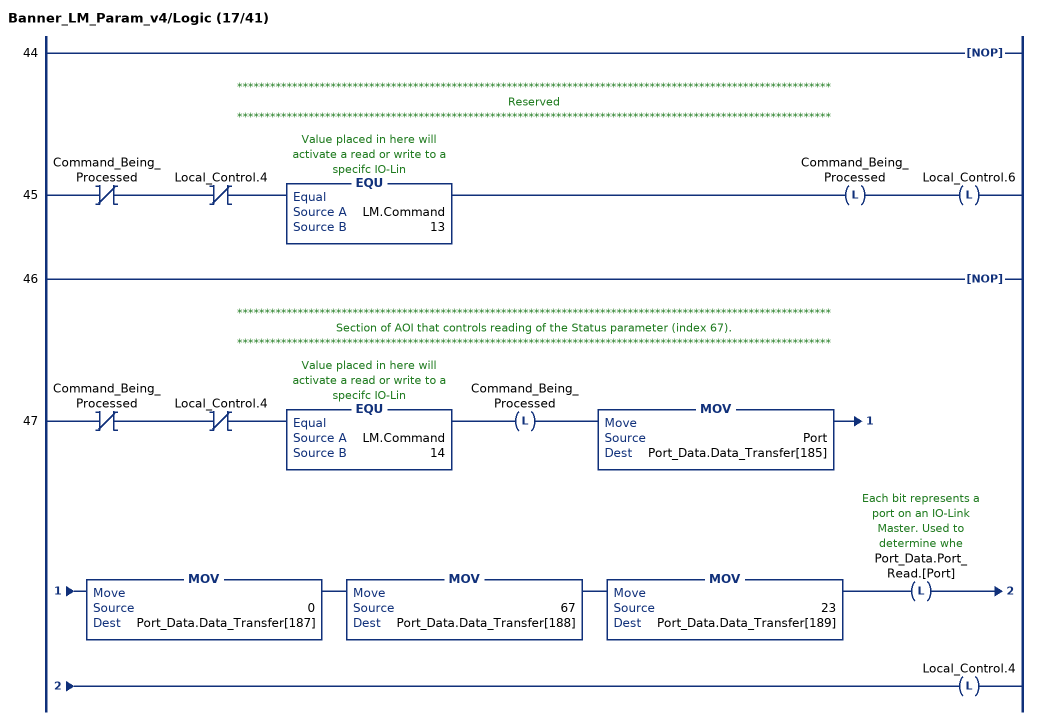
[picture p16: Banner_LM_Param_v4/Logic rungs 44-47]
   44: NOP();
   // ************************************************************************************************************
   // Reserved
   // ************************************************************************************************************
   45: XIO(Command_Being_Processed)XIO(Local_Control.4)EQU(LM.Command,13)OTL(Command_Being_Processed)OTL(Local_Control.6);
   46: NOP();
   // ************************************************************************************************************
   // Section of AOI that controls reading of the Status parameter (index 67).
   // ************************************************************************************************************
   47: XIO(Command_Being_Processed)XIO(Local_Control.4)EQU(LM.Command,14)OTL(Command_Being_Processed)MOV(Port,Port_Data.Data_Transfer[185])MOV(0,Port_Data.Data_Transfer[187])MOV(67,Port_Data.Data_Transfer[188])MOV(23,Port_Data.Data_Transfer[189])OTL(Port_Data.Port_Read.[Port])OTL(Local_Control.4);
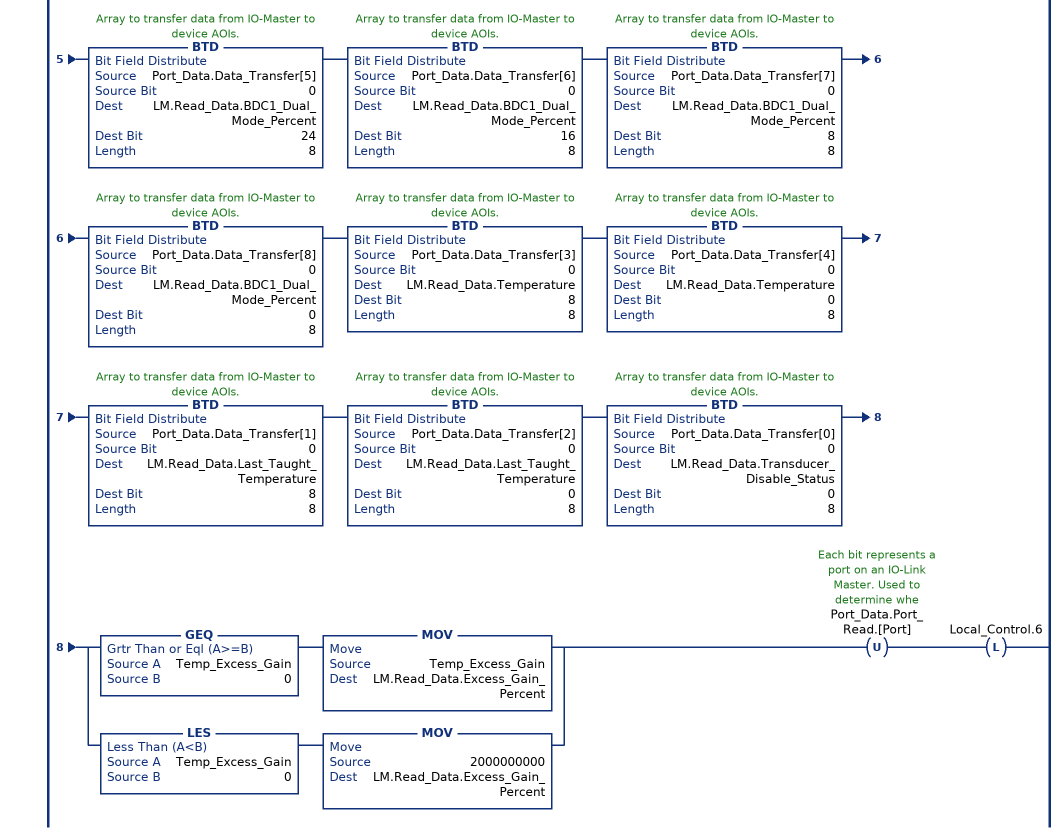
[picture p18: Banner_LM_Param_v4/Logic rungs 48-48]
   48: XIC(Local_Control.5)XIO(Local_Control.6)EQU(LM.Command,14)BTD(Port_Data.Data_Transfer[19],0,LM.Read_Data.Measurement_Distance,24,8)BTD(Port_Data.Data_Transfer[20],0,LM.Read_Data.Measurement_Distance,16,8)BTD(Port_Data.Data_Transfer[21],0,LM.Read_Data.Measurement_Distance,8,8)BTD(Port_Data.Data_Transfer[22],0,LM.Read_Data.Measurement_Distance,0,8)BTD(Port_Data.Data_Transfer[15],0,Temp_Excess_Gain,24,8)BTD(Port_Data.Data_Transfer[16],0,Temp_Excess_Gain,16,8)BTD(Port_Data.Data_Transfer[17],0,Temp_Excess_Gain,8,8)BTD(Port_Data.Data_Transfer[18],0,Temp_Excess_Gain,0,8)BTD(Port_Data.Data_Transfer[14],0,LM.Read_Data.Stability,0,8)BTD(Port_Data.Data_Transfer[13],0,LM.Read_Data.Laser_Fault_Status,0,8)BTD(Port_Data.Data_Transfer[9],0,LM.Read_Data.Analog_Output_Value,24,8)BTD(Port_Data.Data_Transfer[10],0,LM.Read_Data.Analog_Output_Value,16,8)BTD(Port_Data.Data_Transfer[11],0,LM.Read_Data.Analog_Output_Value,8,8)BTD(Port_Data.Data_Transfer[12],0,LM.Read_Data.Analog_Output_Value,0,8)BTD(Port_Data.Data_Transfer[5],0,LM.Read_Data.BDC1_Dual_Mode_Percent,24,8)BTD(Port_Data.Data_Transfer[6],0,LM.Read_Data.BDC1_Dual_Mode_Percent,16,8)BTD(Port_Data.Data_Transfer[7],0,LM.Read_Data.BDC1_Dual_Mode_Percent,8,8)BTD(Port_Data.Data_Transfer[8],0,LM.Read_Data.BDC1_Dual_Mode_Percent,0,8)BTD(Port_Data.Data_Transfer[3],0,LM.Read_Data.Temperature,8,8)BTD(Port_Data.Data_Transfer[4],0,LM.Read_Data.Temperature,0,8)BTD(Port_Data.Data_Transfer[1],0,LM.Read_Data.Last_Taught_Temperature,8,8)BTD(Port_Data.Data_Transfer[2],0,LM.Read_Data.Last_Taught_Temperature,0,8)BTD(Port_Data.Data_Transfer[0],0,LM.Read_Data.Transducer_Disable_Status,0,8)[GEQ(Temp_Excess_Gain,0) MOV(Temp_Excess_Gain,LM.Read_Data.Excess_Gain_Percent) ,LES(Temp_Excess_Gain,0) MOV(2000000000,LM.Read_Data.Excess_Gain_Percent) ]OTU(Port_Data.Port_Read.[Port])OTL(Local_Control.6);
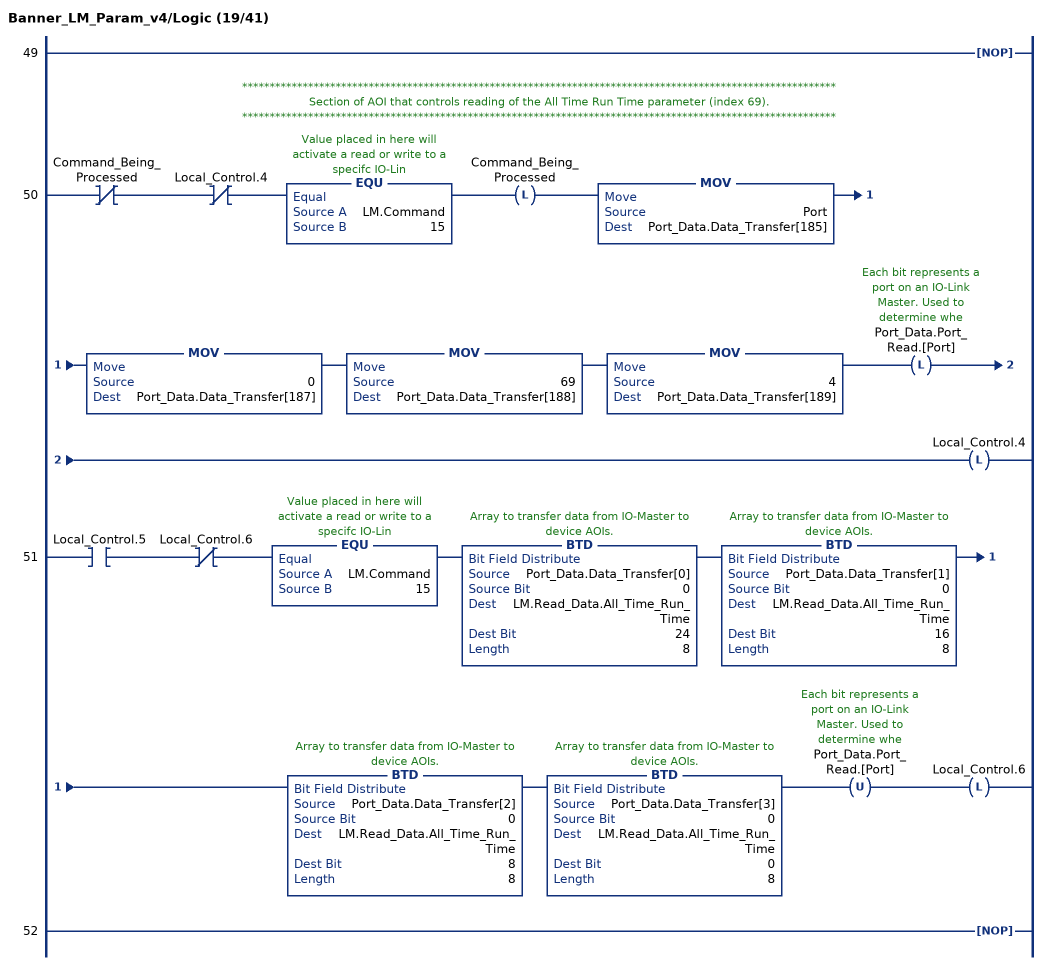
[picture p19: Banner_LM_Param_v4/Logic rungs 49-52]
   49: NOP();
   // ************************************************************************************************************
   // Section of AOI that controls reading of the All Time Run Time parameter (index 69).
   // ************************************************************************************************************
   50: XIO(Command_Being_Processed)XIO(Local_Control.4)EQU(LM.Command,15)OTL(Command_Being_Processed)MOV(Port,Port_Data.Data_Transfer[185])MOV(0,Port_Data.Data_Transfer[187])MOV(69,Port_Data.Data_Transfer[188])MOV(4,Port_Data.Data_Transfer[189])OTL(Port_Data.Port_Read.[Port])OTL(Local_Control.4);
   51: XIC(Local_Control.5)XIO(Local_Control.6)EQU(LM.Command,15)BTD(Port_Data.Data_Transfer[0],0,LM.Read_Data.All_Time_Run_Time,24,8)BTD(Port_Data.Data_Transfer[1],0,LM.Read_Data.All_Time_Run_Time,16,8)BTD(Port_Data.Data_Transfer[2],0,LM.Read_Data.All_Time_Run_Time,8,8)BTD(Port_Data.Data_Transfer[3],0,LM.Read_Data.All_Time_Run_Time,0,8)OTU(Port_Data.Port_Read.[Port])OTL(Local_Control.6);
   52: NOP();
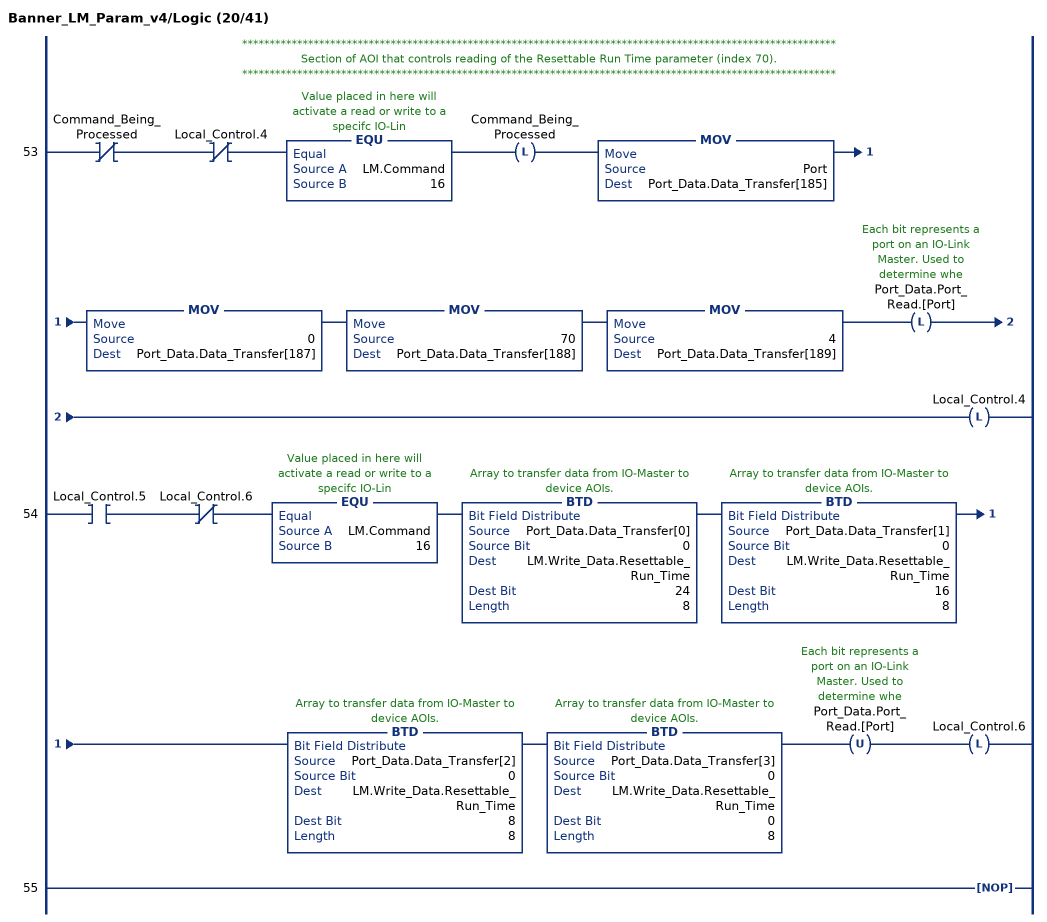
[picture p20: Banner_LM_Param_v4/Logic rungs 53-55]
   // ************************************************************************************************************
   // Section of AOI that controls reading of the Resettable Run Time parameter (index 70).
   // ************************************************************************************************************
   53: XIO(Command_Being_Processed)XIO(Local_Control.4)EQU(LM.Command,16)OTL(Command_Being_Processed)MOV(Port,Port_Data.Data_Transfer[185])MOV(0,Port_Data.Data_Transfer[187])MOV(70,Port_Data.Data_Transfer[188])MOV(4,Port_Data.Data_Transfer[189])OTL(Port_Data.Port_Read.[Port])OTL(Local_Control.4);
   54: XIC(Local_Control.5)XIO(Local_Control.6)EQU(LM.Command,16)BTD(Port_Data.Data_Transfer[0],0,LM.Write_Data.Resettable_Run_Time,24,8)BTD(Port_Data.Data_Transfer[1],0,LM.Write_Data.Resettable_Run_Time,16,8)BTD(Port_Data.Data_Transfer[2],0,LM.Write_Data.Resettable_Run_Time,8,8)BTD(Port_Data.Data_Transfer[3],0,LM.Write_Data.Resettable_Run_Time,0,8)OTU(Port_Data.Port_Read.[Port])OTL(Local_Control.6);
   55: NOP();
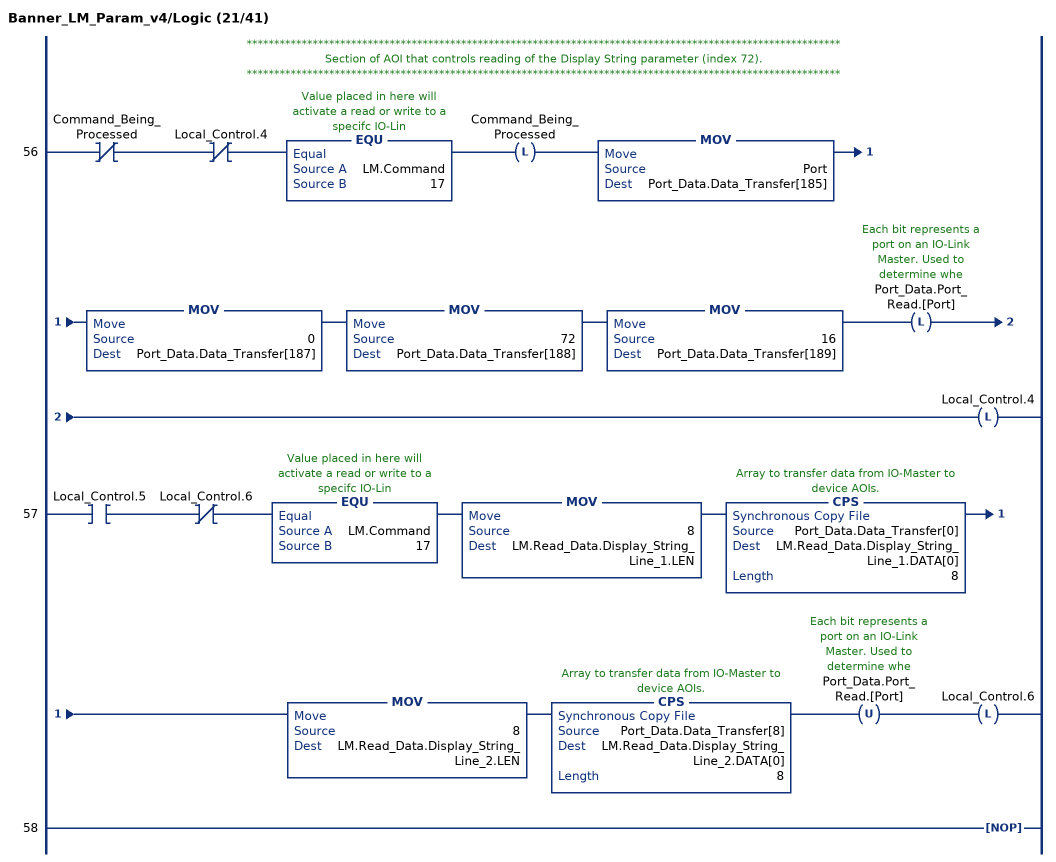
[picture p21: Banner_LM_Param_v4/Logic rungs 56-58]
   // ************************************************************************************************************
   // Section of AOI that controls reading of the Display String parameter (index 72).
   // ************************************************************************************************************
   56: XIO(Command_Being_Processed)XIO(Local_Control.4)EQU(LM.Command,17)OTL(Command_Being_Processed)MOV(Port,Port_Data.Data_Transfer[185])MOV(0,Port_Data.Data_Transfer[187])MOV(72,Port_Data.Data_Transfer[188])MOV(16,Port_Data.Data_Transfer[189])OTL(Port_Data.Port_Read.[Port])OTL(Local_Control.4);
   57: XIC(Local_Control.5)XIO(Local_Control.6)EQU(LM.Command,17)MOV(8,LM.Read_Data.Display_String_Line_1.LEN)CPS(Port_Data.Data_Transfer[0],LM.Read_Data.Display_String_Line_1.DATA[0],8)MOV(8,LM.Read_Data.Display_String_Line_2.LEN)CPS(Port_Data.Data_Transfer[8],LM.Read_Data.Display_String_Line_2.DATA[0],8)OTU(Port_Data.Port_Read.[Port])OTL(Local_Control.6);
   58: NOP();
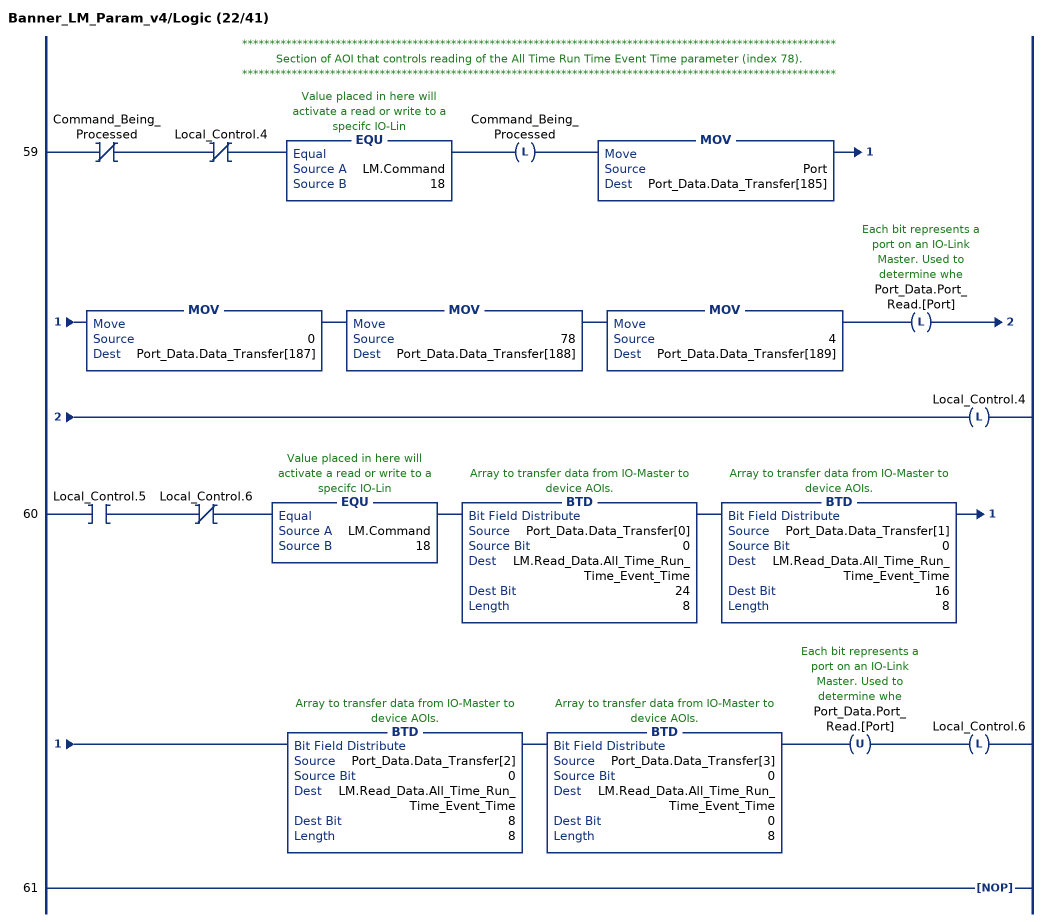
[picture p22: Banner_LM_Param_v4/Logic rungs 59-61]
   // ************************************************************************************************************
   // Section of AOI that controls reading of the All Time Run Time Event Time parameter (index 78).
   // ************************************************************************************************************
   59: XIO(Command_Being_Processed)XIO(Local_Control.4)EQU(LM.Command,18)OTL(Command_Being_Processed)MOV(Port,Port_Data.Data_Transfer[185])MOV(0,Port_Data.Data_Transfer[187])MOV(78,Port_Data.Data_Transfer[188])MOV(4,Port_Data.Data_Transfer[189])OTL(Port_Data.Port_Read.[Port])OTL(Local_Control.4);
   60: XIC(Local_Control.5)XIO(Local_Control.6)EQU(LM.Command,18)BTD(Port_Data.Data_Transfer[0],0,LM.Read_Data.All_Time_Run_Time_Event_Time,24,8)BTD(Port_Data.Data_Transfer[1],0,LM.Read_Data.All_Time_Run_Time_Event_Time,16,8)BTD(Port_Data.Data_Transfer[2],0,LM.Read_Data.All_Time_Run_Time_Event_Time,8,8)BTD(Port_Data.Data_Transfer[3],0,LM.Read_Data.All_Time_Run_Time_Event_Time,0,8)OTU(Port_Data.Port_Read.[Port])OTL(Local_Control.6);
   61: NOP();
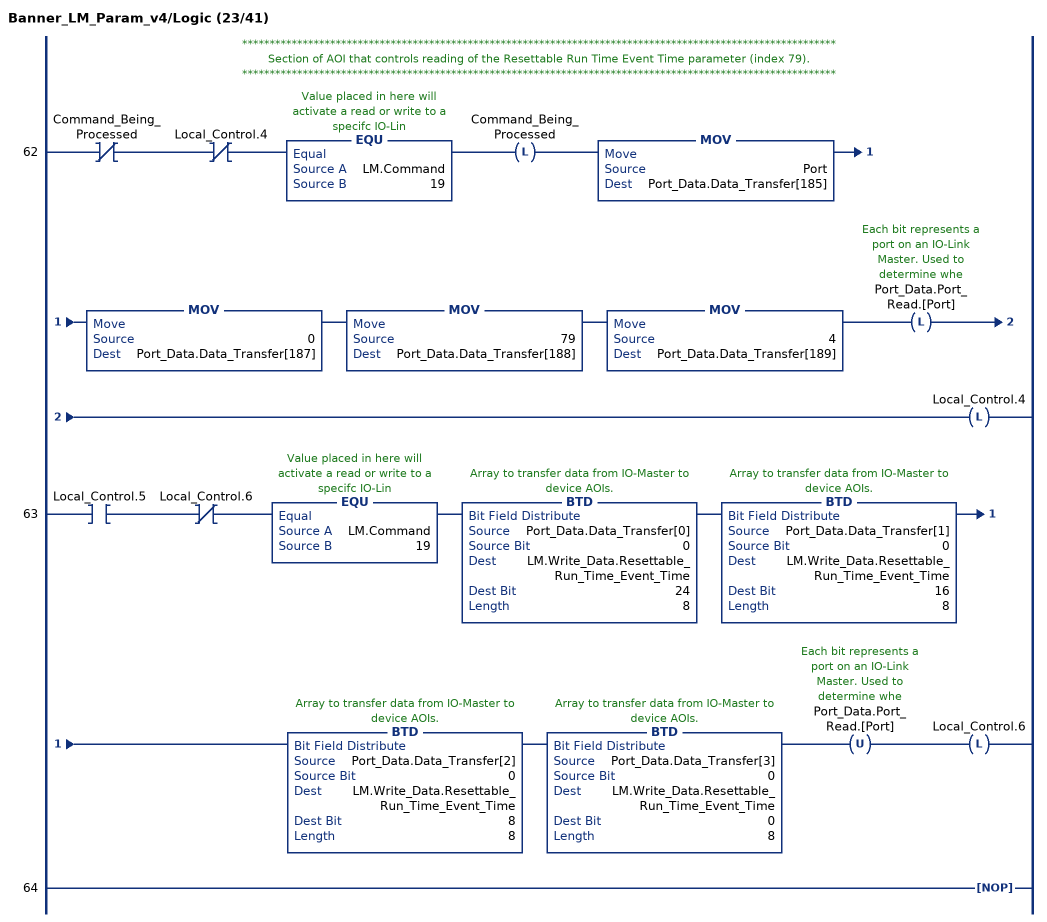
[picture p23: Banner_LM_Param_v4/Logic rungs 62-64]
   // ************************************************************************************************************
   // Section of AOI that controls reading of the Resettable Run Time Event Time parameter (index 79).
   // ************************************************************************************************************
   62: XIO(Command_Being_Processed)XIO(Local_Control.4)EQU(LM.Command,19)OTL(Command_Being_Processed)MOV(Port,Port_Data.Data_Transfer[185])MOV(0,Port_Data.Data_Transfer[187])MOV(79,Port_Data.Data_Transfer[188])MOV(4,Port_Data.Data_Transfer[189])OTL(Port_Data.Port_Read.[Port])OTL(Local_Control.4);
   63: XIC(Local_Control.5)XIO(Local_Control.6)EQU(LM.Command,19)BTD(Port_Data.Data_Transfer[0],0,LM.Write_Data.Resettable_Run_Time_Event_Time,24,8)BTD(Port_Data.Data_Transfer[1],0,LM.Write_Data.Resettable_Run_Time_Event_Time,16,8)BTD(Port_Data.Data_Transfer[2],0,LM.Write_Data.Resettable_Run_Time_Event_Time,8,8)BTD(Port_Data.Data_Transfer[3],0,LM.Write_Data.Resettable_Run_Time_Event_Time,0,8)OTU(Port_Data.Port_Read.[Port])OTL(Local_Control.6);
   64: NOP();
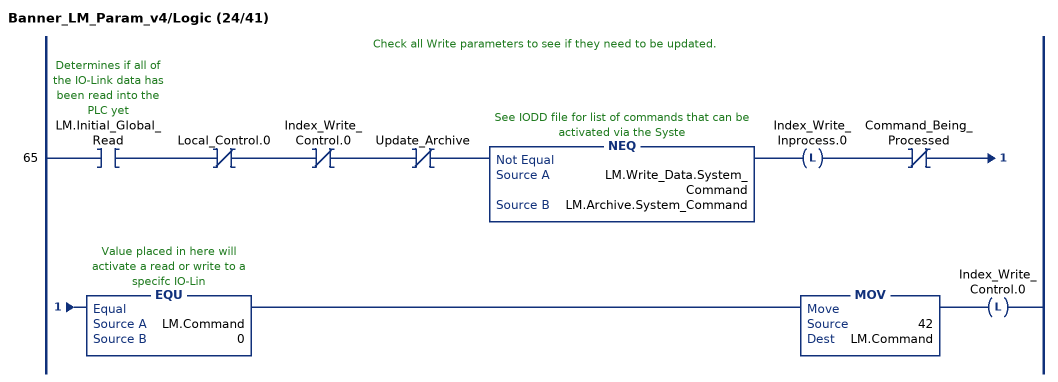
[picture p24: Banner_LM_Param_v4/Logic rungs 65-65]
   // Check all Write parameters to see if they need to be updated.
   65: XIC(LM.Initial_Global_Read)XIO(Local_Control.0)XIO(Index_Write_Control.0)XIO(Update_Archive)NEQ(LM.Write_Data.System_Command,LM.Archive.System_Command)OTL(Index_Write_Inprocess.0)XIO(Command_Being_Processed)EQU(LM.Command,0)MOV(42,LM.Command)OTL(Index_Write_Control.0);
